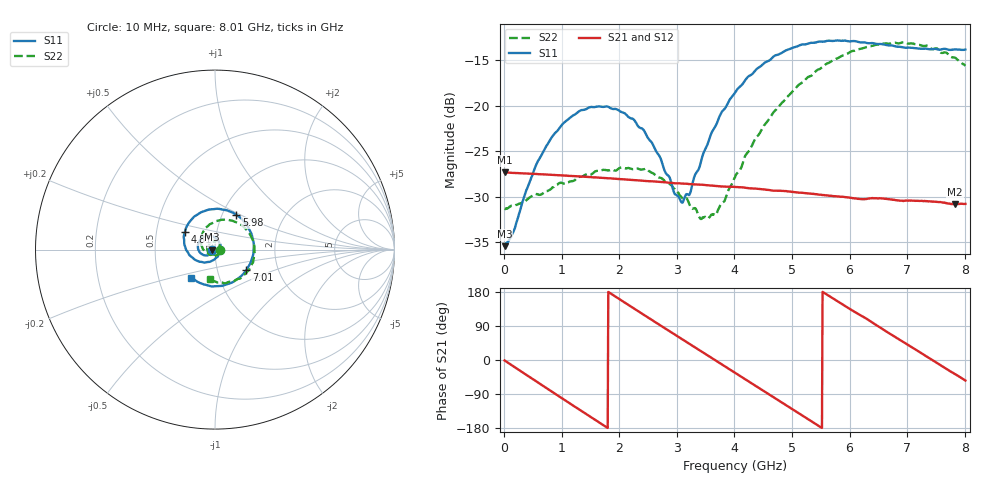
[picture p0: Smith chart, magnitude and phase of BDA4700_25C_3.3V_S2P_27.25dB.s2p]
!Agilent Technologies,E5071B,MY42404982,A.09.10
!Date: Mon Oct 20 18:14:31 2025
!Data & Calibration Information:
!Freq	S11:SOLT2(ON)	S21:SOLT2(ON)	S12:SOLT2(ON)	S22:SOLT2(ON)
# Hz S RI R 50
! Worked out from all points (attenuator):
!   801 points, 10 MHz to 8.01 GHz, reference 50 ohm
!   highest |S21| = -27.31 dB at 20 MHz (marker M1); lowest = -30.8 dB at 7.83 GHz (marker M2)
!   lowest |S11| = -35.4 dB at 10 MHz (marker M3), VSWR 1.03, Z = 48.3 - j0.1 ohm
!   |S11| at or under -10 dB: start of sweep to end of sweep
!   |S22| runs from -32.5 to -13.0 dB; largest |S21 - S12| = 0.0005
!   S11 on the Smith chart (normalised r, x): 10 MHz: 0.97, -0.00; 4.81 GHz: 0.70, +0.15; 5.98 GHz: 1.16, +0.47; 7.01 GHz: 1.38, -0.33; 8.01 GHz: 0.74, -0.24
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1e7  -0.0169 -0.00103  0.0431 -0.000937  0.0431 -0.000966  0.0271 -0.000803
2e7  -0.0172 -0.00164  0.0431 -0.00164  0.043 -0.00172  0.027 -0.00105
1.6e8  -0.0177 -0.00976  0.041 -0.0121  0.041 -0.0121  0.0272 -0.00767
5.3e8  -0.0345 -0.029  0.0251 -0.034  0.0251 -0.034  0.0168 -0.028
7.3e8  -0.0501 -0.0326  0.0119 -0.0402  0.0119 -0.0402  0.00412 -0.0336
1.35e9  -0.0947 0.00413  -0.0289 -0.0289  -0.0288 -0.0289  -0.0365 -0.0182
2.08e9  -0.0536 0.0742  -0.0352 0.0179  -0.0352 0.0178  -0.0302 0.0338
2.68e9  0.0183 0.0508  -0.0031 0.0381  -0.00318 0.0381  0.0129 0.0384
2.96e9  0.0302 0.0129  0.0143 0.0347  0.0143 0.0347  0.026 0.0232
3.1e9  0.0283 -0.00773  0.022 0.0302  0.0218 0.0303  0.0287 0.0118
3.23e9  0.0214 -0.0252  0.0277 0.0247  0.0278 0.0246  0.028 0.00286
3.55e9  -0.0161 -0.0616  0.0359 0.00679  0.036 0.00676  0.0131 -0.0202
3.7e9  -0.042 -0.0691  0.0361 -0.00235  0.0361 -0.00243  0.000455 -0.026
4.01e9  -0.1008 -0.0615  0.0298 -0.0198  0.0298 -0.0197  -0.031 -0.026
4.81e9  -0.1671 0.0996  -0.0122 -0.0318  -0.012 -0.0319  -0.0774 0.0676
5.35e9  -0.0704 0.2107  -0.0314 -0.00957  -0.0313 -0.0097  -0.0162 0.1468
5.98e9  0.1184 0.1932  -0.0229 0.0214  -0.0231 0.0212  0.126 0.149
6.68e9  0.215 -0.00783  0.00994 0.029  0.00999 0.029  0.2193 0.000484
7.01e9  0.1754 -0.1135  0.0228 0.0196  0.0229 0.0194  0.2016 -0.0878
7.45e9  0.0508 -0.1991  0.0297 -0.000811  0.0298 -0.000795  0.113 -0.1706
7.83e9  -0.079 -0.1885  0.0229 -0.0174  0.023 -0.0174  0.0139 -0.1834
8.01e9  -0.131 -0.1564  0.0169 -0.0234  0.017 -0.0233  -0.0303 -0.1634
